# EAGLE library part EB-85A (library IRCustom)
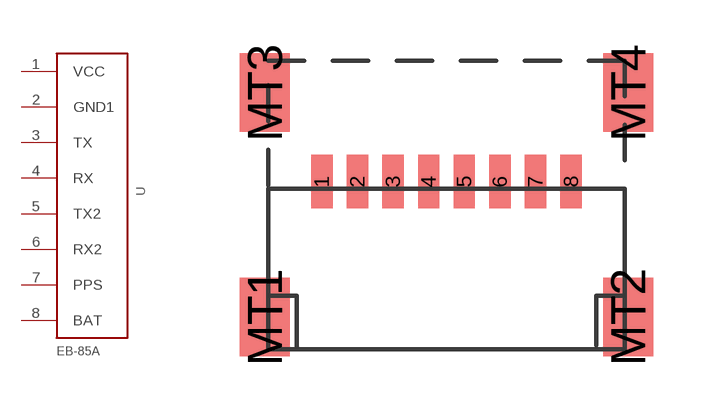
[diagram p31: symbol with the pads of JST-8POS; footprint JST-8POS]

Designator prefix -

## EB-85A  [JST-8POS]
1  VCC  sup
2  GND1  sup
3  TX  out
4  RX  in
5  TX2  out
6  RX2  in
7  PPS  out
8  BAT  sup

## Footprint JST-8POS (pad centres in mm)
smd 0.6 x 1.5: 1 -3.5,0.2; 2 -2.5,0.2; 3 -1.5,0.2; 4 -0.5,0.2; 5 0.5,0.2; 6 1.5,0.2; 7 2.5,0.2; 8 3.5,0.2
smd 1.4 x 2.2: MT1 -5.1,-3.6; MT2 5.1,-3.6; MT3 -5.1,2.7; MT4 5.1,2.7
